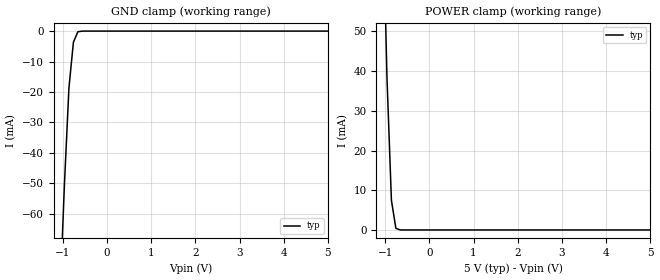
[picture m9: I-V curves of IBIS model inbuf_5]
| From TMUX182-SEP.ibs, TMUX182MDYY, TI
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| inbuf_5
[Model]   inbuf_5
Model_type   Input
Vinl = 0.8
Vinh = 1.35
|   typ   min   max
C_comp   6.362683e-13   NA   NA
[Voltage Range]   5   NA   NA
[Temperature Range]   27   NA   NA
[Power Clamp Reference]   5   NA   NA
[GND Clamp Reference]   0   NA   NA
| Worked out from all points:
|   GND clamp passes 1 mA (typ) near -0.68 V on its own axis
|   POWER clamp passes 1 mA (typ) near -0.77 V on its own axis
[GND Clamp]
|   Voltage   I(typ)   I(min)   I(max)
-5V       -2.674A    NA         NA
-1.061V   -87.09mA   NA         NA
-959.6mV  -50.28mA   NA         NA
-858.6mV  -18.75mA   NA         NA
-757.6mV  -3.722mA   NA         NA
-656.6mV  -214.5uA   NA         NA
-454.5mV  -852.8nA   NA         NA
5V        464.6nA    NA         NA
[POWER Clamp]
|   Voltage   I(typ)   I(min)   I(max)
-5V       3.151A     NA         NA
-1.061V   85.92mA    NA         NA
-959.6mV  38.53mA    NA         NA
-858.6mV  7.472mA    NA         NA
-757.6mV  394uA      NA         NA
-656.6mV  10.62uA    NA         NA
-555.6mV  703.5nA    NA         NA
5V        -6.944pA   NA         NA
